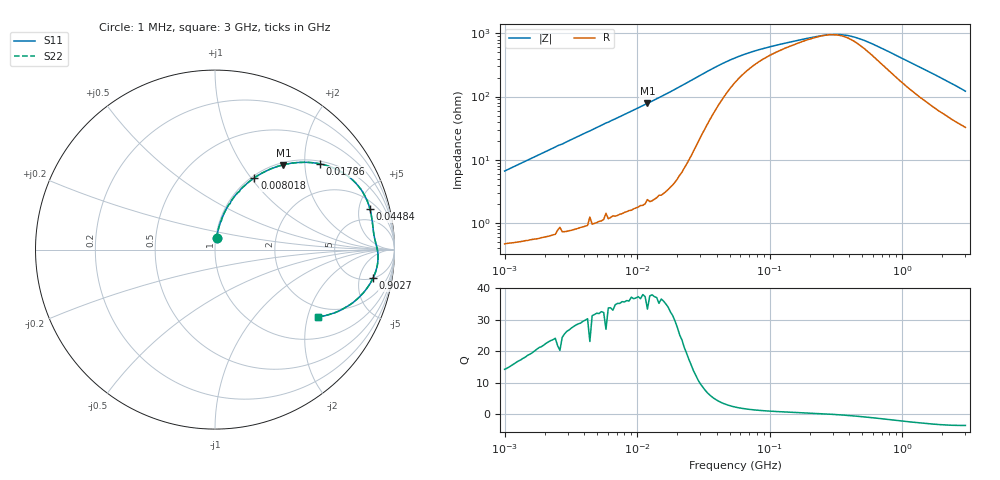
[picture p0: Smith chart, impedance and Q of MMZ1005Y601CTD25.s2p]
! S-Parameter Data Generated by TDK Corporation
! Copyright(C) 2025 TDK Corporation.
! All Rights Reserved.
! TDK P/N: MMZ1005Y601CTD25 (Chip Bead)
! Property: |Z|=600ohm at 100MHz
! Size(LxWxT): 1x0.5x0.5mm
! Model Type: s2p (Touchstone File Format Version 1.0)
! Frequency: DC=Yes Start=1MHz Stop=3000MHz 202points Log-sweep
! Model Generated on Feb. 6, 2025
! Terms and conditions regarding TDK Simulation Models:
! 1)This simulation model is being provided solely for informational
!  purposes. Please refer to the specifications of the products in
!  terms of detailed characteristics of such products.
! 2)In no event shall TDK Corporation of any of its subsidiaries be
!  liable for any loss or damage arising, directly or indirectly,
!  from any information contained in this simulation model, including,
!  but not limited to loss or damages arising from any inaccuracies,
!  omissions or errors in connection with such information.
! 3)Any and all copyrights on this simulation model are owned by
!  TDK Corporation.  Duplication or redistribution of this simulation
!  model without prior written permission from TDK Corporation
!  is prohibited.
! 4)This simulation model is subject to any modification or change
!  without any prior notice.
! 5)Neither TDK Corporation nor any of its subsidiaries shall make any
!  warranty, express or implied, including but not limited to the
!  correctness, implied warranties of merchantability and fitness for
!  a particular purpose with respect to this simulation models.
! 6)The use of this simulation model shall be deemed to have consented
!  to the terms and conditions hereof.
! Port Assignments:
!  1 ---@@@--- 2
! Applicable Conditions:
!  Temperature = 25 degC
!  DC Bias Current = 0 A
!  Small Signal Operation
# Hz S MA R 50
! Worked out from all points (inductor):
!   201 points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, 1 MHz to 3 GHz, reference 50 ohm
!   read as one part in series: L = 1.05 uH near 1.041 MHz
!   highest Q = 37.5 at 11.96 MHz (marker M1), where L = 1.04 uH
!   self-resonance near 274.9 MHz
!   S11 on the Smith chart (normalised r, x): 1 MHz: 1.01, +0.13; 8.018 MHz: 1.03, +1.04; 17.86 MHz: 1.07, +2.38; 44.84 MHz: 2.93, +6.50; 902.7 MHz: 5.02, -8.00; 3 GHz: 1.65, -2.34
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1000000  0.0656 82.2  0.9933 -3.8  0.9933 -3.8  0.0656 82.2
2055611  0.1331 79.8  0.9852 -7.6  0.9852 -7.6  0.1331 79.8
3900413  0.2445 73.9  0.9614 -14.1  0.9614 -14.1  0.2445 73.9
6058321  0.3616 67.1  0.9217 -21.2  0.9217 -21.2  0.3616 67.1
8017732  0.456 61.3  0.8773 -27.1  0.8773 -27.1  0.456 61.3
1.196486e7  0.606 51.0  0.7775 -37.3  0.7775 -37.3  0.606 51.0
1.461624e7  0.6831 45.3  0.7112 -43.1  0.7112 -43.1  0.6831 45.3
1.785516e7  0.7549 39.2  0.633 -49.0  0.633 -49.0  0.7549 39.2
2.181181e7  0.8155 33.0  0.5451 -54.6  0.5451 -54.6  0.8155 33.0
2.886629e7  0.8703 24.6  0.4187 -60.1  0.4187 -60.1  0.8703 24.6
4.483659e7  0.8927 14.6  0.2631 -58.8  0.2631 -58.8  0.8927 14.6
5.477226e7  0.8911 11.5  0.2178 -54.4  0.2178 -54.4  0.8911 11.5
8.854986e7  0.8885 6.5  0.155 -40.8  0.155 -40.8  0.8885 6.5
2.136344e8  0.8996 1.4  0.1031 -12.5  0.1031 -12.5  0.8996 1.4
2.827291e8  0.9051 -0.2  0.09491 1.6  0.09491 1.6  0.9051 -0.2
3.894533e8  0.9094 -2.3  0.09812 21.5  0.09812 21.5  0.9094 -2.3
5.154121e8  0.9097 -4.5  0.117 37.3  0.117 37.3  0.9097 -4.5
8.005644e8  0.9003 -8.8  0.1771 51.4  0.1771 51.4  0.9003 -8.8
9.0272e8  0.8943 -10.3  0.1998 53.1  0.1998 53.1  0.8943 -10.3
1.243477e9  0.871 -14.7  0.2718 54.6  0.2718 54.6  0.871 -14.7
1.782824e9  0.8233 -21.0  0.3752 51.9  0.3752 51.9  0.8233 -21.0
3e9  0.6876 -33.0  0.5653 41.5  0.5653 41.5  0.6876 -33.0
